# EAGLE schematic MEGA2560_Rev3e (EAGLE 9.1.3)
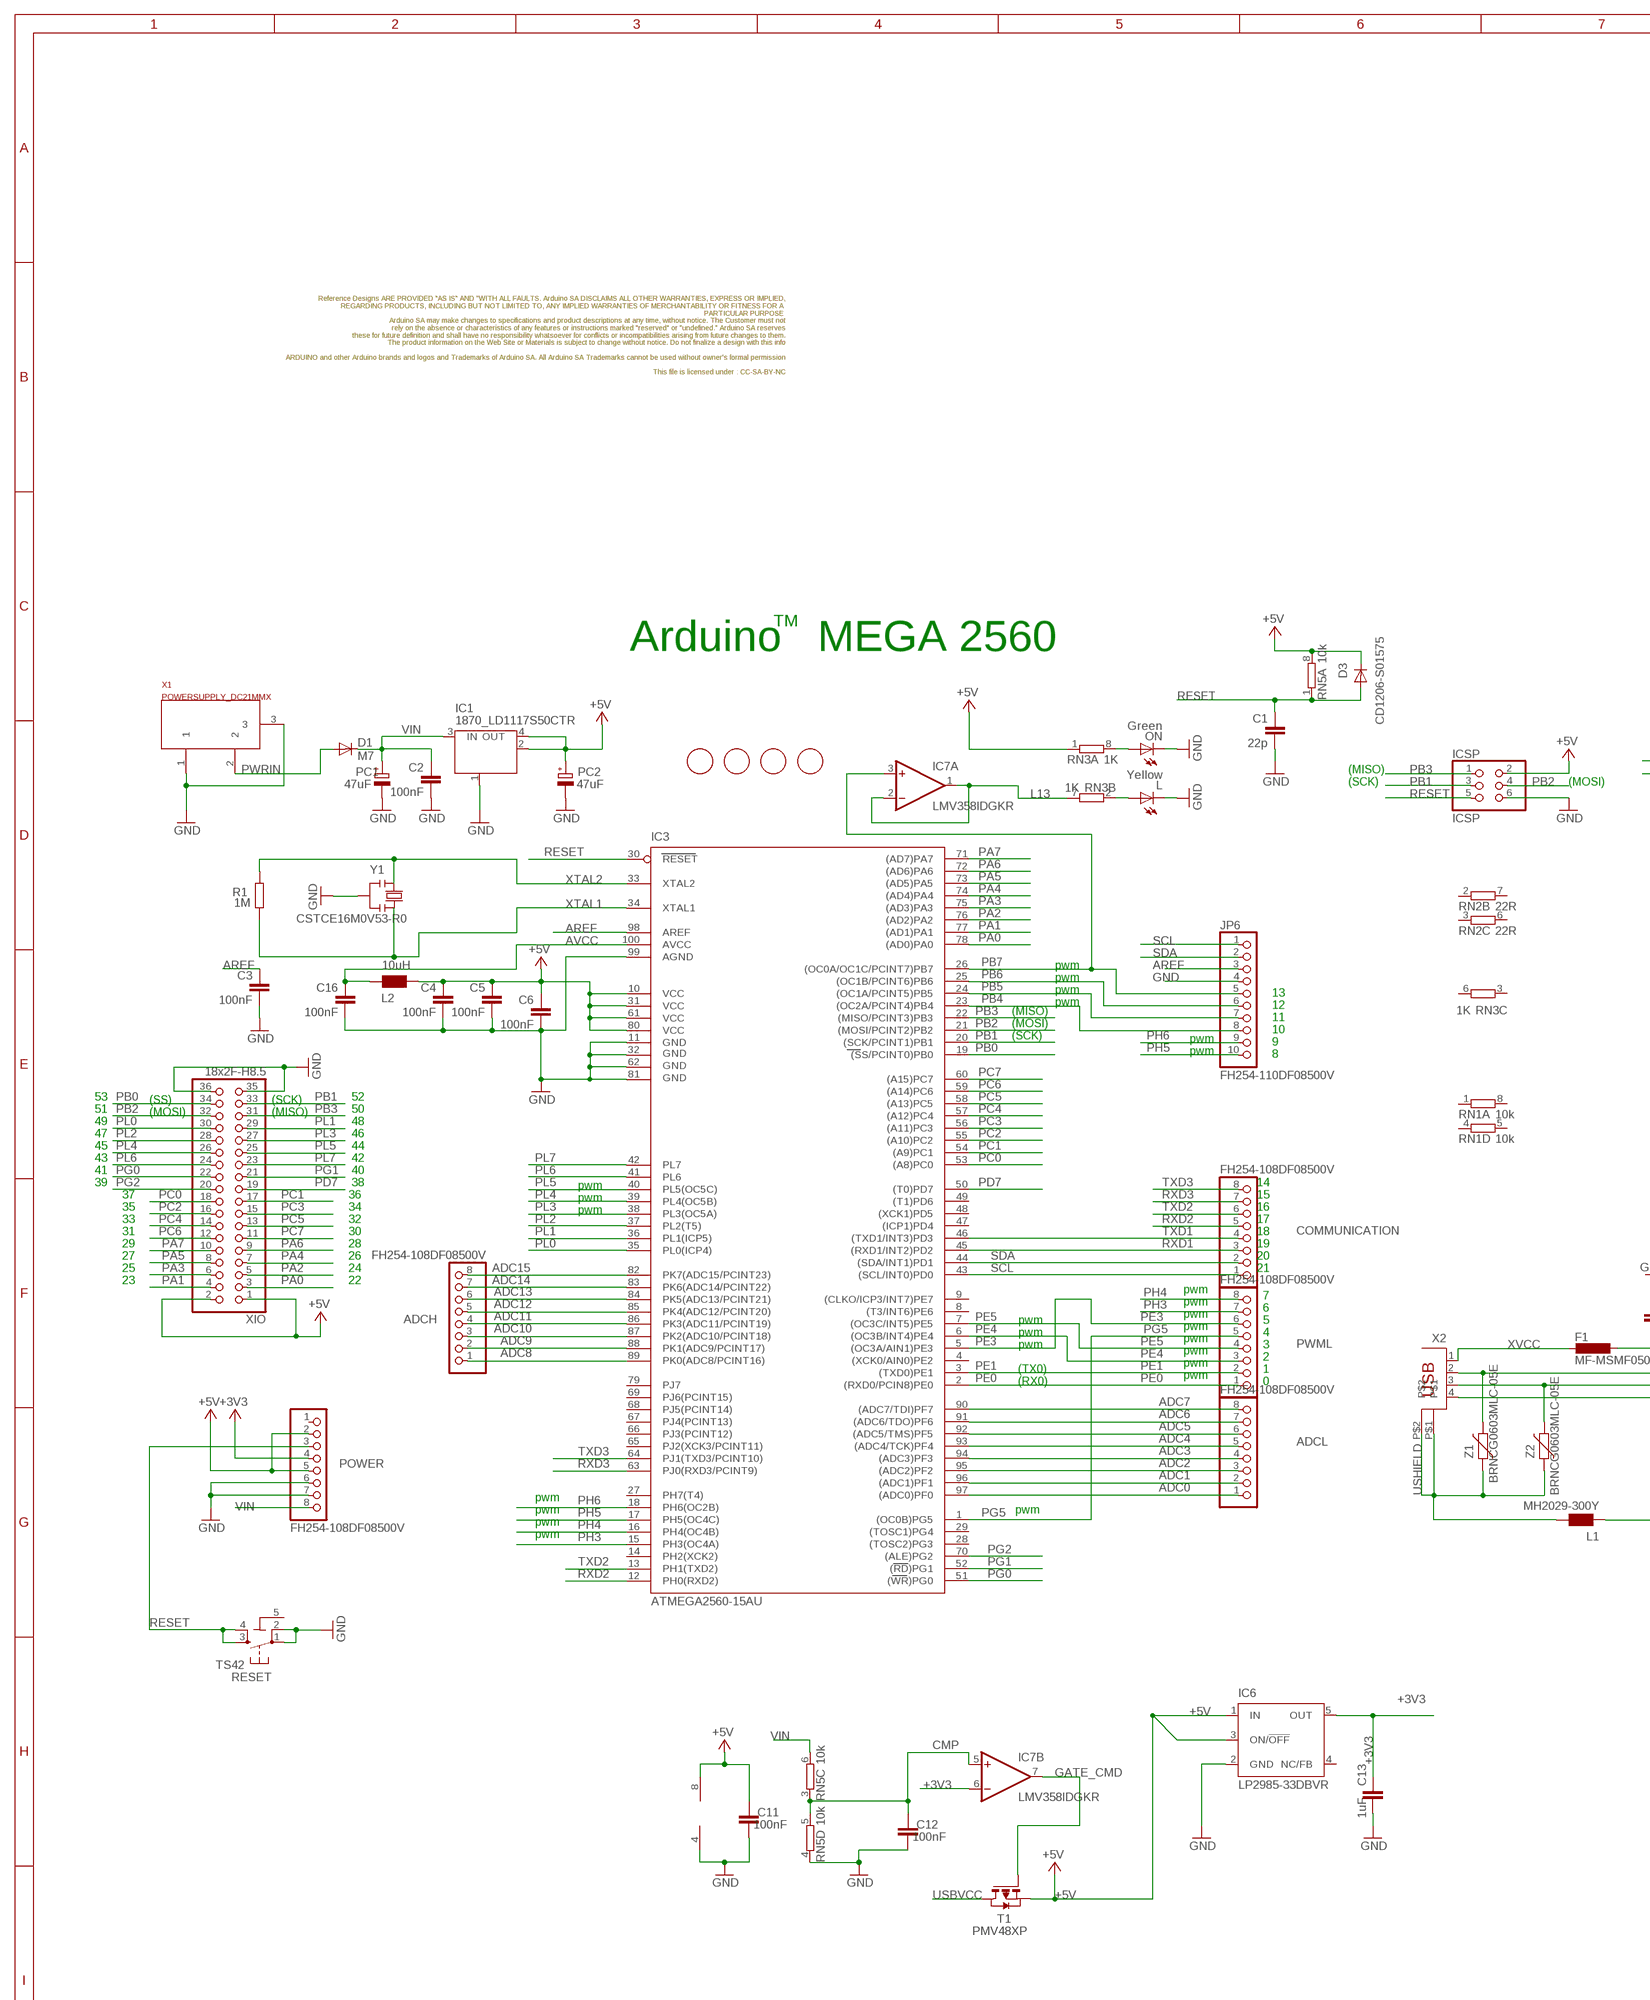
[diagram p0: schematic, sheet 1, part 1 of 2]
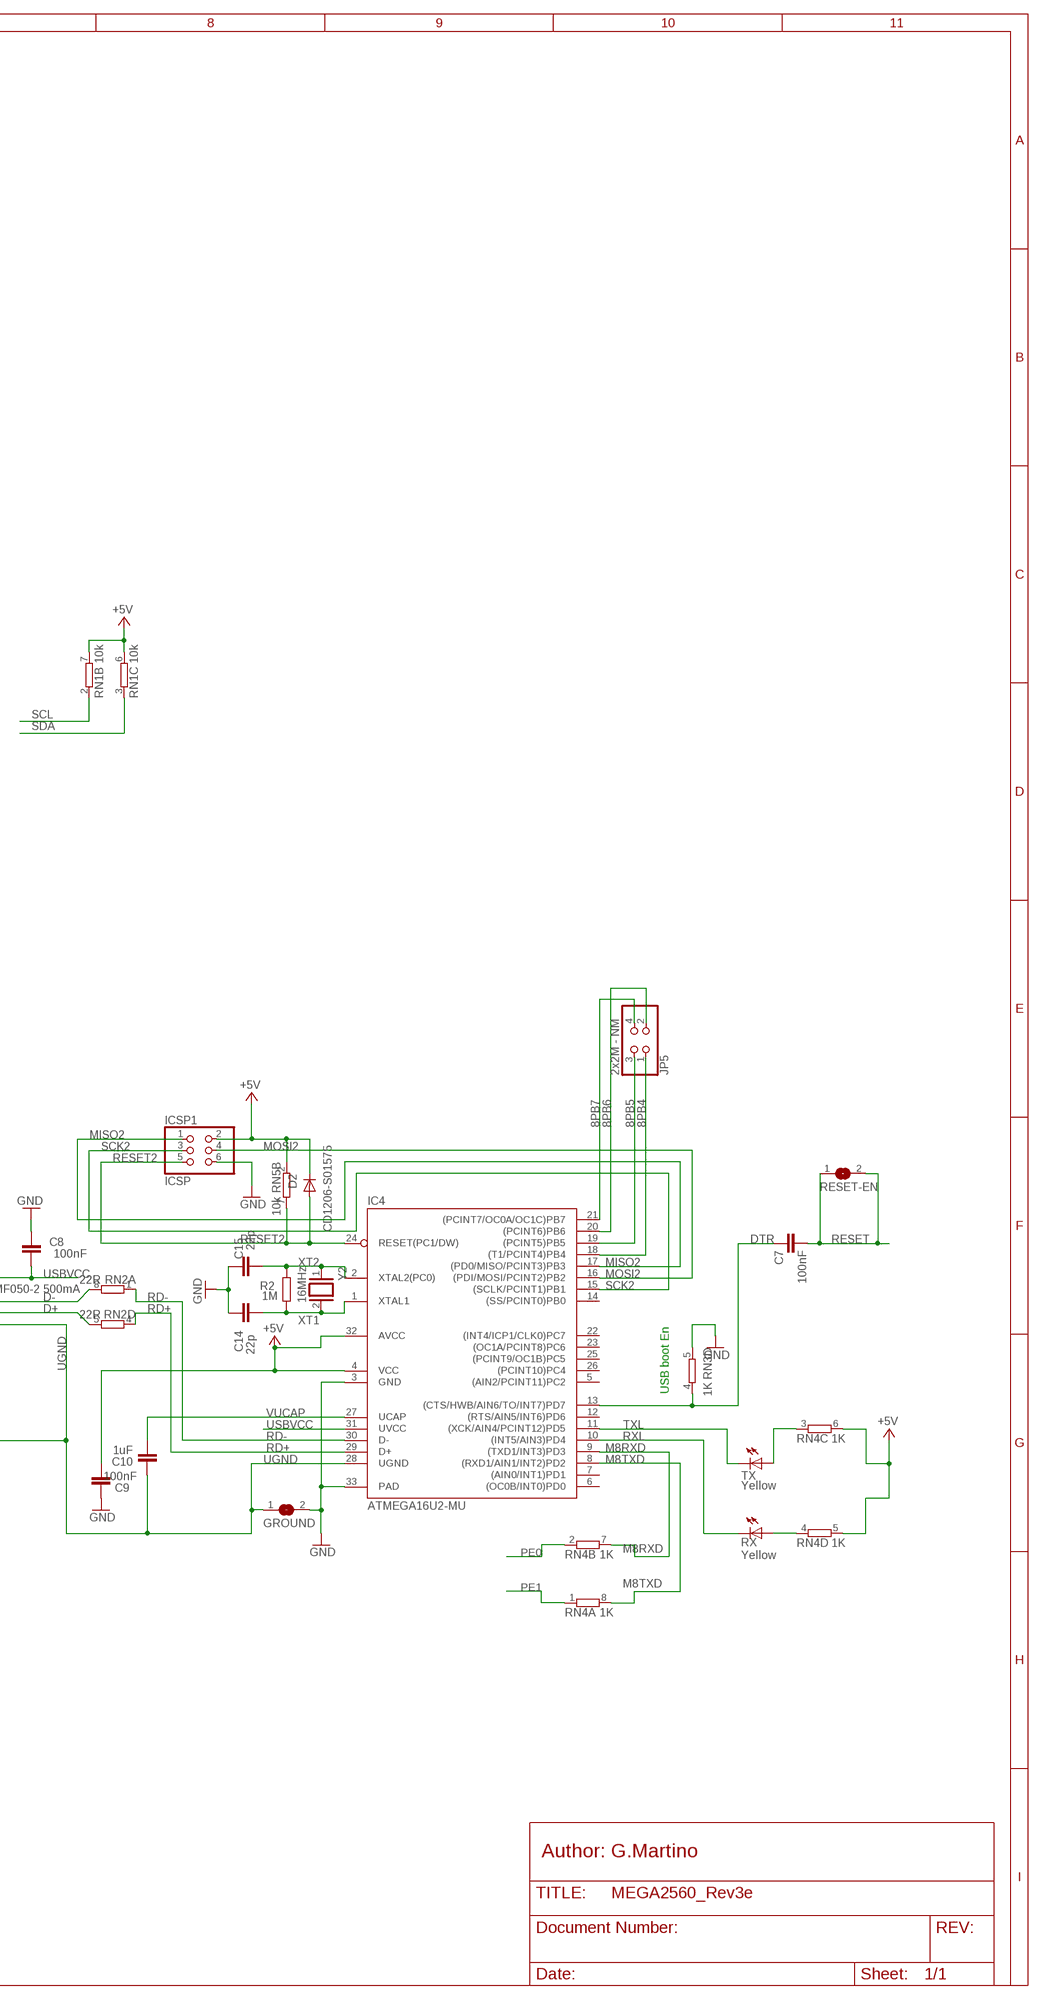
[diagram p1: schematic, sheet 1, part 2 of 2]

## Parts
ADCH  FH254-108DF08500V  0058_FH254-108DF08500V  [1X08]
ADCL  FH254-108DF08500V  0058_FH254-108DF08500V  [1X08]
C1  22p  0014_22PF_0603  [C0603-ROUND]
C2  100nF  0015_100NF_0603  [C0603-ROUND]
C3  100nF  0015_100NF_0603  [C0603-ROUND]
C4  100nF  0015_100NF_0603  [C0603-ROUND]
C5  100nF  0015_100NF_0603  [C0603-ROUND]
C6  100nF  0015_100NF_0603  [C0603-ROUND]
C7  100nF  0015_100NF_0603  [C0603-ROUND]
C8  100nF  0015_100NF_0603  [C0603-ROUND]
C9  100nF  0015_100NF_0603  [C0603-ROUND]
C10  1uF  0006_1UF_0603/GRM188R61E105KA12D  [C0603-ROUND]
C11  100nF  0015_100NF_0603  [C0603-ROUND]
C12  100nF  0015_100NF_0603  [C0603-ROUND]
C13  1uF  0006_1UF_0603/GRM188R61E105KA12D  [C0603-ROUND]
C14  22p  0014_22PF_0603  [C0603-ROUND]
C15  22p  0014_22PF_0603  [C0603-ROUND]
C16  100nF  0015_100NF_0603  [C0603-ROUND]
COMMUNICATION  FH254-108DF08500V  0058_FH254-108DF08500V  [1X08]
D1  M7  0020_M7  [SMB]
D2  CD1206-S01575  0012_CD1206-S01575  [MINIMELF]
D3  CD1206-S01575  0012_CD1206-S01575  [MINIMELF]
F1  MF-MSMF050-2 500mA  0002_MF-MSMF050-2  [L1812]
FD1  FIDUCIALMOUNT  [FIDUCIA-MOUNT]
FD2  FIDUCIALMOUNT  [FIDUCIA-MOUNT]
FD3  FIDUCIALMOUNT  [FIDUCIA-MOUNT]
FD4  FIDUCIALMOUNT  [FIDUCIA-MOUNT]
FRAME2  TEXTTEXT_BRDSCH  [FRAME]
GROUND  SJ  [SJ]
IC1  1870_LD1117S50CTR  [LINEAR_SOT223]
IC3  ATMEGA2560-15AU  0023_ATMEGA2560-16AU  [TQFP100]
IC4  ATMEGA16U2-MU  0007_ATMEGA16U2-MUR  [MLF32]
IC6  LP2985-33DBVR  0008_TEXLP2985-33DBVR  [SOT23-DBV]
IC7  LMV358IDGKR  0021_LMV358IDGKR  [MSOP08]
ICSP  ICSP  0114_PH254-203DF118A00V  [2X03]
ICSP1  ICSP  0114_PH254-203DF118A00V  [2X03]
JP5  2x2M - NM  PINHD-2X2  [2X02]
JP6  FH254-110DF08500V  1216_FH254-110DF08500T30  [1X10]
L  Yellow  0044_KPT-2012YC  [CHIPLED_0805]
L1  MH2029-300Y  0001_BLM21PG300SN1D_/_MH2029-300Y  [0805]
L2  10uH  0715_CV201210-100K  [0805]
ON  Green  0043_KPT-2012SGC  [CHIPLED_0805]
PC1  47uF  0113_47UF  [PANASONIC_D]
PC2  47uF  0113_47UF  [PANASONIC_D]
POWER  FH254-108DF08500V  1217_FH254-108DF08500T21  [1X08]
PWML  FH254-108DF08500V  1218_FH254-108DF08500T20  [1X08]
R1  1M  0004_0603_1M  [R0603-ROUND]
R2  1M  0004_0603_1M  [R0603-ROUND]
RESET  TS42  0946_TS42031-160W-TR-7260  [TS42]
RESET-EN  SJ  [SJ]
RN1  10k  0016_064R_10K_/_CAY16-103J4LF  [CAY16]
RN2  22R  0003_064R_22R_/_CAY16-220J4LF  [CAY16]
RN3  1K  0005_064R_1K_/_CAY16-102J4LF  [CAY16]
RN4  1K  0005_064R_1K_/_CAY16-102J4LF  [CAY16]
RN5  10k  0016_064R_10K_/_CAY16-103J4LF  [CAY16]
RX  Yellow  0044_KPT-2012YC  [CHIPLED_0805]
T1  PMV48XP  0297_PMV48XP  [SOT-23]
TX  Yellow  0044_KPT-2012YC  [CHIPLED_0805]
X1  POWERSUPPLY_DC21MMX  [POWERSUPPLY_DC-21MM]
X2  0056_USB-B-S-RA-WT-SPCC  [PN61729]
XIO  18x2F-H8.5  0060_FH254-218DF08500V  [2X18]
Y1  CSTCE16M0V53-R0  0011_CSTCE16M0V53-R0  [RESONATOR]
Y2  16MHz  0019_P011052006_16M  [QS]
Z1  BRNCG0603MLC-05E  0010_BRNCG0603MLC-05E  [CT/CN0603]
Z2  BRNCG0603MLC-05E  0010_BRNCG0603MLC-05E  [CT/CN0603]

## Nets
8PB4: IC4.18((T1/PCINT4)PB4) JP5.1
8PB5: IC4.19((PCINT5)PB5) JP5.3
8PB6: IC4.20((PCINT6)PB6) JP5.2
8PB7: IC4.21((PCINT7/OC0A/OC1C)PB7) JP5.4
+3V3 [power]: C13.2 IC6.5(OUT) IC7.6(B:-IN) POWER.4
+5V [power usb]: C4.1 C5.1 C6.1 C9.1 C11.2 D2.C D3.C IC1.2(OUT) IC1.4(OUT) IC3.10(VCC) IC3.31(VCC1) IC3.61(VCC2) IC3.80(VCC3) IC4.4(VCC) IC4.32(AVCC) IC6.1(IN) IC6.3(ON/!OFF) IC7.8(P:V+) ICSP1.2 ICSP.2 L2.2 PC2.+ POWER.2 POWER.5 RN1.6 RN1.7 RN3.1 RN4.5 RN4.6 RN5.2 RN5.8 T1.2(S) XIO.1 XIO.2
ADC0: ADCL.1 IC3.97((ADC0)PF0)
ADC1: ADCL.2 IC3.96((ADC1)PF1)
ADC2: ADCL.3 IC3.95((ADC2)PF2)
ADC3: ADCL.4 IC3.94((ADC3)PF3)
ADC4: ADCL.5 IC3.93((ADC4/TCK)PF4)
ADC5: ADCL.6 IC3.92((ADC5/TMS)PF5)
ADC6: ADCL.7 IC3.91((ADC6/TDO)PF6)
ADC7: ADCL.8 IC3.90((ADC7/TDI)PF7)
ADC8: ADCH.1 IC3.89(PK0(ADC8/PCINT16))
ADC9: ADCH.2 IC3.88(PK1(ADC9/PCINT17))
ADC10: ADCH.3 IC3.87(PK2(ADC10/PCINT18))
ADC11: ADCH.4 IC3.86(PK3(ADC11/PCINT19))
ADC12: ADCH.5 IC3.85(PK4(ADC12/PCINT20))
ADC13: ADCH.6 IC3.84(PK5(ADC13/PCINT21))
ADC14: ADCH.7 IC3.83(PK6(ADC14/PCINT22))
ADC15: ADCH.8 IC3.82(PK7(ADC15/PCINT23))
AREF: C3.1 IC3.98(AREF) JP6.3
AVCC [power usb]: C16.1 IC3.100(AVCC) L2.1
CMP: C12.2 IC7.5(B:+IN) RN5.3 RN5.5
D+: RN2.5 X2.3 Z2.2
D-: RN2.8 X2.2 Z1.2
DTR: C7.1 IC4.13((CTS/HWB/AIN6/TO/INT7)PD7) RN3.4
GATE_CMD: IC7.7(B:OUT) T1.3(G)
GND [gnd]: C1.2 C2.2 C3.2 C4.2 C5.2 C6.2 C8.2 C9.2 C11.1 C12.1 C13.1 C14.2 C15.2 C16.2 GROUND.2 IC1.1(GND/ADJ) IC3.11(GND) IC3.32(GND1) IC3.62(GND2) IC3.81(GND3) IC3.99(AGND) IC4.3(GND) IC4.33(PAD) IC6.2(GND) IC7.4(P:V-) ICSP1.6 ICSP.6 JP6.4 L.C ON.C PC1.- PC2.- POWER.6 POWER.7 RESET.1 RESET.2 RN3.5 RN5.4 X1.1 X1.3 XIO.35 XIO.36 Y1.2
L13: IC7.1(A:OUT) IC7.2(A:-IN) RN3.7
M8RXD: IC4.9((TXD1/INT3)PD3) RN4.7
M8TXD: IC4.8((RXD1/AIN1/INT2)PD2) RN4.8
MISO2: IC4.17((PD0/MISO/PCINT3)PB3) ICSP1.1
MOSI2: IC4.16((PDI/MOSI/PCINT2)PB2) ICSP1.4
N$2: L.A RN3.2
N$3: ON.A RN3.8
N$54: RN4.4 RX.A
N$55: RN4.3 TX.A
PA0: IC3.78((AD0)PA0) XIO.3
PA1: IC3.77((AD1)PA1) XIO.4
PA2: IC3.76((AD2)PA2) XIO.5
PA3: IC3.75((AD3)PA3) XIO.6
PA4: IC3.74((AD4)PA4) XIO.7
PA5: IC3.73((AD5)PA5) XIO.8
PA6: IC3.72((AD6)PA6) XIO.9
PA7: IC3.71((AD7)PA7) XIO.10
PB0: IC3.19((SS/PCINT0)PB0) XIO.34
PB1: IC3.20((SCK/PCINT1)PB1) ICSP.3 XIO.33
PB2: IC3.21((MOSI/PCINT2)PB2) ICSP.4 XIO.32
PB3: IC3.22((MISO/PCINT3)PB3) ICSP.1 XIO.31
PB4: IC3.23((OC2A/PCINT4)PB4) JP6.8
PB5: IC3.24((OC1A/PCINT5)PB5) JP6.7
PB6: IC3.25((OC1B/PCINT6)PB6) JP6.6
PB7: IC3.26((OC0A/OC1C/PCINT7)PB7) IC7.3(A:+IN) JP6.5
PC0: IC3.53((A8)PC0) XIO.18
PC1: IC3.54((A9)PC1) XIO.17
PC2: IC3.55((A10)PC2) XIO.16
PC3: IC3.56((A11)PC3) XIO.15
PC4: IC3.57((A12)PC4) XIO.14
PC5: IC3.58((A13)PC5) XIO.13
PC6: IC3.59((A14)PC6) XIO.12
PC7: IC3.60((A15)PC7) XIO.11
PD7: IC3.50((T0)PD7) XIO.19
PE0: IC3.2((RXD0/PCIN8)PE0) PWML.1 RN4.2
PE1: IC3.3((TXD0)PE1) PWML.2 RN4.1
PE3: IC3.5((OC3A/AIN1)PE3) PWML.6
PE4: IC3.6((OC3B/INT4)PE4) PWML.3
PE5: IC3.7((OC3C/INT5)PE5) PWML.4
PG0: IC3.51((WR)PG0) XIO.22
PG1: IC3.52((RD)PG1) XIO.21
PG2: IC3.70((ALE)PG2) XIO.20
PG5: IC3.1((OC0B)PG5) PWML.5
PH3: IC3.15(PH3(OC4A)) PWML.7
PH4: IC3.16(PH4(OC4B)) PWML.8
PH5: IC3.17(PH5(OC4C)) JP6.10
PH6: IC3.18(PH6(OC2B)) JP6.9
PL0: IC3.35(PL0(ICP4)) XIO.30
PL1: IC3.36(PL1(ICP5)) XIO.29
PL2: IC3.37(PL2(T5)) XIO.28
PL3: IC3.38(PL3(OC5A)) XIO.27
PL4: IC3.39(PL4(OC5B)) XIO.26
PL5: IC3.40(PL5(OC5C)) XIO.25
PL6: IC3.41(PL6) XIO.24
PL7: IC3.42(PL7) XIO.23
PWRIN [power]: D1.A X1.2
RD+: IC4.29(D+) RN2.4
RD-: IC4.30(D-) RN2.1
RESET: C1.1 C7.2 D3.A IC3.30(RESET) ICSP.5 POWER.3 RESET-EN.1 RESET-EN.2 RESET.3 RESET.4 RN5.1
RESET2: D2.A IC4.24(RESET(PC1/DW)) ICSP1.5 RN5.7
RXD1: COMMUNICATION.3 IC3.45((RXD1/INT2)PD2)
RXD2: COMMUNICATION.5 IC3.12(PH0(RXD2))
RXD3: COMMUNICATION.7 IC3.63(PJ0(RXD3/PCINT9))
RXL: IC4.10((INT5/AIN3)PD4) RX.C
SCK2: IC4.15((SCLK/PCINT1)PB1) ICSP1.3
SCL: COMMUNICATION.1 IC3.43((SCL/INT0)PD0) JP6.1 RN1.2
SDA: COMMUNICATION.2 IC3.44((SDA/INT1)PD1) JP6.2 RN1.3
TXD1: COMMUNICATION.4 IC3.46((TXD1/INT3)PD3)
TXD2: COMMUNICATION.6 IC3.13(PH1(TXD2))
TXD3: COMMUNICATION.8 IC3.64(PJ1(TXD3/PCINT10))
TXL: IC4.11((XCK/AIN4/PCINT12)PD5) TX.C
UGND [gnd]: C10.2 GROUND.1 IC4.28(UGND) L1.1 X2.4
USBVCC [power usb]: C8.1 F1.1 IC4.31(UVCC) T1.1(D)
USHIELD [gnd]: L1.2 X2.P$1 X2.P$2 Z1.1 Z2.1
VIN [power]: C2.1 D1.C IC1.3(IN) PC1.+ POWER.8 RN5.6
VUCAP: C10.1 IC4.27(UCAP)
XT1: C14.1 IC4.1(XTAL1) R2.1 Y2.2
XT2: C15.1 IC4.2(XTAL2(PC0)) R2.2 Y2.1
XTAL1: IC3.34(XTAL1) R1.1 Y1.3
XTAL2: IC3.33(XTAL2) R1.2 Y1.1
XVCC [power usb]: F1.2 X2.1
Unconnected: IC3.4((XCK0/AIN0)PE2) IC3.8((T3/INT6)PE6) IC3.9((CLKO/ICP3/INT7)PE7) IC3.14(PH2(XCK2)) IC3.27(PH7(T4)) IC3.28((TOSC2)PG3) IC3.29((TOSC1)PG4) IC3.47((ICP1)PD4) IC3.48((XCK1)PD5) IC3.49((T1)PD6) IC3.65(PJ2(XCK3/PCINT11)) IC3.66(PJ3(PCINT12)) IC3.67(PJ4(PCINT13)) IC3.68(PJ5(PCINT14)) IC3.69(PJ6(PCINT15)) IC3.79(PJ7) IC4.5((AIN2/PCINT11)PC2) IC4.6((OC0B/INT0)PD0) IC4.7((AIN0/INT1)PD1) IC4.12((RTS/AIN5/INT6)PD6) IC4.14((SS/PCINT0)PB0) IC4.22((INT4/ICP1/CLK0)PC7) IC4.23((OC1A/PCINT8)PC6) IC4.25((PCINT9/OC1B)PC5) IC4.26((PCINT10)PC4) IC6.4(NC/FB) POWER.1 RN1.1 RN1.4 RN1.5 RN1.8 RN2.2 RN2.3 RN2.6 RN2.7 RN3.3 RN3.6

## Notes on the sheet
- TM
- Arduino   MEGA 2560
- (MISO)
- (SCK) | (MOSI)
- pwm
- pwm
- pwm | 13
- pwm | 12
- (MISO)
- 11
- (MOSI)
- 10
- (SCK) | pwm
- 9
- pwm | 8
- 53 | (SS) | (SCK) | 52
- 51 | (MOSI) | (MISO) | 50
- 49 | 48
- 47 | 46
- 45 | 44
- 43 | 42
- 41 | 40
- 39 | 38 | pwm | 14
- 37 | 36 | pwm | 15
- 35 | 34 | pwm | 16
- 33 | 32 | 17
- 31 | 30 | 18
- 29 | 28 | 19
- 27 | 26 | 20
- 25 | 24 | 21
- 23 | 22
- pwm
- 7
- pwm
- 6
- pwm
- pwm | 5
- pwm
- pwm | 4
- pwm
- pwm | 3
- pwm
- 2
- pwm
- (TX0) | 1
- pwm
- (RX0) | 0
- USB boot En
- pwm
- pwm | pwm
- pwm
- pwm
- Author: G.Martino

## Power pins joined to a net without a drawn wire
5-GND: RESET.5(5-GND)

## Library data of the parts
ADCH ADCL COMMUNICATION = Connettori:0058_FH254-108DF08500V: Female Connector strip for Arduino bases - 8x1 F V h 8,5 p2,54mm; MONTHLY_USAGE: _____; PART_NUMBER: FH254-108DF08500V; PRICE: _____; SUPPLIER: _____; TYPE: Connettori
C1 C14 C15 = Condensatori:0014_22PF_0603: 22pF 0603; CASE: 0603; MONTHLY_USAGE: _____; PART_NUMBER: 22pF_0603; PRICE: _____; SUPPLIER: _____; TYPE: Condensatori
C2-C9 C11 C12 C16 = Condensatori:0015_100NF_0603: 100nF 0603 50V; CASE: 0603; MONTHLY_USAGE: _____; PART_NUMBER: cl10b104kbnc; PRICE: _____; SUPPLIER: _____; TYPE: Condensatori
C10 C13 = Condensatori:0006_1UF_0603/GRM188R61E105KA12D: 1uF 0603; CASE: 0603; MONTHLY_USAGE: _____; PART_NUMBER: 1uF_0603/GRM188R61E105KA12D; PRICE: _____; SUPPLIER: _____; TYPE: Condensatori
D1 = Diodi:0020_M7: 1.0A 40V SURFACE MOUNT GLASS PASSIVATED RECTIFIER M7; CASE: SMA; MONTHLY_USAGE: _____; PART_NUMBER: M7; PRICE: _____; SUPPLIER: _____; TYPE: Diodi
D2 D3 = Diodi:0012_CD1206-S01575: small-signal high-speed Switching Diodes CD1206; CASE: 1206; MONTHLY_USAGE: _____; PART_NUMBER: CD1206-S01575; PRICE: _____; SUPPLIER: _____; TYPE: Diodi
F1 = Protezione:0002_MF-MSMF050-2: 500 mA Multifuse � Polyfuse; MONTHLY_USAGE: _____; PART_NUMBER: MF-MSMF050-2; PRICE: _____; SUPPLIER: _____; TYPE: Protezione
FD1-FD4 = SmartPrj:FIDUCIALMOUNT
FRAME2 = Arduino-utility:TEXT: TEXT
GROUND RESET-EN = jumper:SJ: SMD solder JUMPER
IC1 = IntegratedCircuits:1870_LD1117S50CTR: Low-dropout linear regulator 5V -LM1117IMPX-5.0; CASE: SOT223; MONTHLY_USAGE: _____; PART_NUMBER: LD1117S50CTR; PRICE: _____; SUPPLIER: _____; TYPE: Circuito_Integrato; VALUE: LD1117S50CTR
IC3 = IntegratedCircuits:0023_ATMEGA2560-16AU: 8-bit Microcontroller with 256K Bytes In-System Programmable Flash - ATMEGA2560-16AU; CASE: TQFP100_14x14; MONTHLY_USAGE: _____; PART_NUMBER: ATMEGA2560-16AU; PRICE: _____; SUPPLIER: _____; TYPE: Circuito_Integrato
IC4 = IntegratedCircuits:0007_ATMEGA16U2-MUR: 8-bit Microcontroller with 16K Bytes of ISP Flash and USB Controller ATMEGA16U2-MUR; CASE: QFN32_5x5; MONTHLY_USAGE: _____; PART_NUMBER: ATMEGA16U2-MUR; PRICE: _____; SUPPLIER: _____; TYPE: Circuito_Integrato
IC6 = IntegratedCircuits:0008_TEXLP2985-33DBVR: 150-mA LOW-NOISE LOW-DROPOUT REGULATOR WITH SHUTDOWN LP2985-33DBVR; CASE: SOT23-5; MONTHLY_USAGE: _____; PART_NUMBER: TEXLP2985-33DBVR; PRICE: _____; SUPPLIER: _____; TYPE: Circuito_Integrato
IC7 = IntegratedCircuits:0021_LMV358IDGKR: Dual low-voltage (2.7 V to 5.5 V), operational amplifiers with rail-to-rail output swing LMV358IDGKR; CASE: MSOP8; MONTHLY_USAGE: _____; PART_NUMBER: LMV358IDGKR; PRICE: _____; SUPPLIER: _____; TYPE: Circuito_Integrato
ICSP ICSP1 = Connettori:0114_PH254-203DF118A00V: 3x2 M V h 8,5 mm p2,54; MONTHLY_USAGE: _____; PART_NUMBER: PH254-203DF118A00V; PRICE: _____; SUPPLIER: _____; TYPE: Connettori
JP5 = SmartPrj:PINHD-2X2: PIN HEADER
JP6 = Connettori:1216_FH254-110DF08500T30: Female Connector strip for Arduino bases - 10x1 F V h 8,5 p2,54 serigrafato STRISCIA VUOTA; MONTHLY_USAGE: _____; PART_NUMBER: FH254-110DF08500T30; PRICE: _____; SUPPLIER: _____; TYPE: Connettori; VALUE: FH254-110DF08500T30
L RX TX = Opto:0044_KPT-2012YC: LED YELLOW - SMD - 0805; MONTHLY_USAGE: _____; PART_NUMBER: KPT-2012YC; PRICE: _____; SUPPLIER: _____; TYPE: Opto
L1 = Protezione:0001_BLM21PG300SN1D_/_MH2029-300Y: BLM21; MONTHLY_USAGE: _____; PART_NUMBER: BLM21PG300SN1D_/_MH2029-300Y; PRICE: _____; SUPPLIER: _____; TYPE: Protezione
L2 = Induttanze:0715_CV201210-100K: 10uH 0805; CASE: 0805; MONTHLY_USAGE: _____; PART_NUMBER: CV201210-100K; PRICE: _____; SUPPLIER: _____; TYPE: Induttanze
ON = Opto:0043_KPT-2012SGC: LED GREEN - SMD-0805; MONTHLY_USAGE: _____; PART_NUMBER: KPT-2012SGC; PRICE: _____; SUPPLIER: _____; TYPE: Opto
PC1 PC2 = Condensatori:0113_47UF: 47uF; MONTHLY_USAGE: _____; PART_NUMBER: 47uF; PRICE: _____; SUPPLIER: _____; TYPE: Condensatori
POWER = Connettori:1217_FH254-108DF08500T21: Female Connector strip for Arduino bases - 8x1 F V h 8,5 p2,54 serigrafato POWER; MONTHLY_USAGE: _____; PART_NUMBER: FH254-108DF08500T21; PRICE: _____; SUPPLIER: _____; TYPE: Connettori; VALUE: FH254-108DF08500T21
PWML = Connettori:1218_FH254-108DF08500T20: Female Connector strip for Arduino bases - 8x1 F V h 8,5 p2,54 serigrafato DIGITAL; MONTHLY_USAGE: _____; PART_NUMBER: FH254-108DF08500T20; PRICE: _____; SUPPLIER: _____; TYPE: Connettori; VALUE: FH254-108DF08500T20
R1 R2 = Resistenze:0004_0603_1M: 1M 0603; CASE: 0603; MONTHLY_USAGE: _____; PART_NUMBER: 0603_1M; PRICE: _____; SUPPLIER: _____; TYPE: Resistenze
RESET = Switches:0946_TS42031-160W-TR-7260: Pushbutton 6x6 Smd - White; MONTHLY_USAGE: _____; PART_NUMBER: IT-1157AHNP-160G-G_GTR; PRICE: _____; SUPPLIER: _____; TYPE: Switches
RN1 RN5 = Resistenze:0016_064R_10K_/_CAY16-103J4LF: 10K 064 R; CASE: SMD_3,2x1,6; MONTHLY_USAGE: _____; PART_NUMBER: 064R_10K_/_CAY16-103J4LF; PRICE: _____; SUPPLIER: _____; TYPE: Resistenze
RN2 = Resistenze:0003_064R_22R_/_CAY16-220J4LF: 22R 064R; CASE: SMD_3,2x1,6; MONTHLY_USAGE: _____; PART_NUMBER: 064R_22R_/_CAY16-220J4LF; PRICE: _____; SUPPLIER: _____; TYPE: Resistenze
RN3 RN4 = Resistenze:0005_064R_1K_/_CAY16-102J4LF: 1K 064R; CASE: SMD_3,2x1,6; MONTHLY_USAGE: _____; PART_NUMBER: 064R_1K_/_CAY16-102J4LF; PRICE: _____; SUPPLIER: _____; TYPE: Resistenze
T1 = Transistors:0297_PMV48XP: 20 V, 3.5 A P-channel Trench MOSFET - PMV48XP; CASE: SOT23; MONTHLY_USAGE: _____; PART_NUMBER: PMV48XP; PRICE: _____; SUPPLIER: _____; TYPE: Transistor
X1 = SmartPrj:POWERSUPPLY_DC21MM
X2 = Connettori:0056_USB-B-S-RA-WT-SPCC: USB - B; MONTHLY_USAGE: _____; PART_NUMBER: USB-B-S-RA-WT-SPCC; PRICE: _____; SUPPLIER: _____; TYPE: Connettori
XIO = Connettori:0060_FH254-218DF08500V: 18x2 F V h 8,5 p2,54; MONTHLY_USAGE: _____; PART_NUMBER: FH254-218DF08500V; PRICE: _____; SUPPLIER: _____; TYPE: Connettori
Y1 = Cristalli:0011_CSTCE16M0V53-R0: 16Mhz - SMD; MONTHLY_USAGE: _____; PART_NUMBER: CSTCE16M0V53-R0; PRICE: _____; SUPPLIER: _____; TYPE: Cristalli
Y2 = Cristalli:0019_P011052006_16M: 16MHz THT; PART_NUMBER: P011052006 16M/FTX16M20S; TYPE: Cristalli
Z1 Z2 = Protezione:0010_BRNCG0603MLC-05E: CG0603MLC-05E; MONTHLY_USAGE: _____; PART_NUMBER: BRNCG0603MLC-05E; PRICE: _____; SUPPLIER: _____; TYPE: Protezione

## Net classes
0 default: width 0.203 mm, drill 0.406 mm, clearance 0.203 mm
1 power: width 0.61 mm, drill 0.406 mm, clearance 0.203 mm
2 gnd: width 0.305 mm, drill 0.406 mm, clearance 0.203 mm
3 power usb: width 0.508 mm, drill 0.406 mm, clearance 0.203 mm

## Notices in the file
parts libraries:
Arduino-utility: Copyright (c) 2016-2017 Arduino LLC. All right reserved.
Arduino-utility: This file is licensed under : CC-SA-BY-NC
